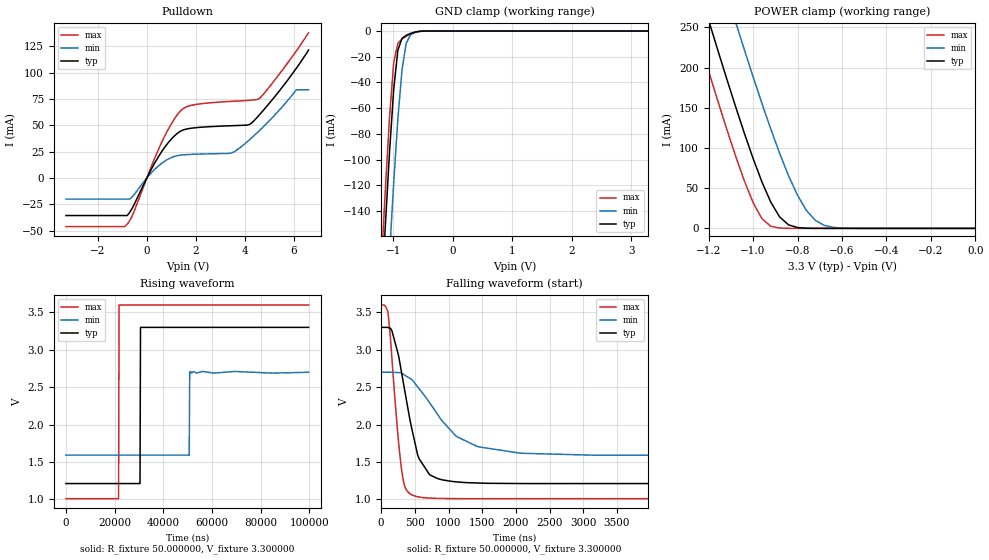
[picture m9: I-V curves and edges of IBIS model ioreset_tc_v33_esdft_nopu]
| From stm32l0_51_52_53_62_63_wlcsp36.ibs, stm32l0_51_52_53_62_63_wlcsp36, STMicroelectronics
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|   Model ioreset_tc_v33_esdft_nopu
[Model]  ioreset_tc_v33_esdft_nopu
Model_type I/O_open_drain
Polarity   Inverting
Enable   Active-High
Vinl =   0.990000V
Vinh =   2.310000V
Vmeas =  1.650000V
Cref =   1.0000000000000001E-7F
Rref =   1.000000k
Vref =   3.300000V
C_comp   1.946100pF   1.923200pF   1.977700pF
[Temperature Range]   25.000000   0.125000k   -40.000000
[Pullup Reference]   3.300000V   2.700000V   3.600000V
[Pulldown Reference]   0.0V   0.0V   0.0V
[POWER Clamp Reference]   3.300000V   2.700000V   3.600000V
[GND Clamp Reference]   0.0V   0.0V   0.0V
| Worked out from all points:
|   slope of the pulldown table from 0 to 0.495 V, typ, clamps not added: 23.6 ohm
|   GND clamp passes 1 mA (typ) near -0.65 V on its own axis
|   POWER clamp passes 1 mA (typ) near -0.80 V on its own axis
|   rising waveform, R_fixture 50.000000, V_fixture 3.300000: 20-80 % time 120ns typ, 119ns min, 120ns max; typ from 1.21 V to 3.3 V
|   falling waveform, R_fixture 50.000000, V_fixture 3.300000: 20-80 % time 267ns typ, 617ns min, 142ns max; typ from 3.3 V to 1.21 V
[Pulldown]
|Voltage   I(typ)   I(min)   I(max)
-3.3V     -35.57mA   -19.98mA   -46.06mA
-900mV    -35.57mA   -19.98mA   -46.06mA
-600mV    -28.81mA   -18.01mA   -36.04mA
600mV     24.81mA    13.84mA    33.52mA
1V        36.95mA    19.4mA     51.38mA
1.4V      44.71mA    21.77mA    64.22mA
1.9V      47.49mA    22.51mA    69.34mA
3.4V      49.55mA    23.44mA    72.65mA
4.2V      50.88mA    36.54mA    73.75mA
4.7V      62.76mA    47.3mA     77.96mA
6.1V      104.1mA    83.7mA     120.5mA
6.6V      121.4mA    83.7mA     137.7mA
[GND_clamp]
|Voltage   I(typ)   I(min)   I(max)
-3.3V     -2.25A     -2.322A    -2.233A
-1.2V     -211.8mA   -294.7mA   -184.2mA
-1.13V    -151mA     -233.2mA   -123.1mA
-1.06V    -94.15mA   -173.8mA   -67.07mA
-990mV    -45.49mA   -118mA     -24.73mA
-920mV    -14.87mA   -68.31mA   -9.524mA
-850mV    -5.685mA   -30.05mA   -6.27mA
-780mV    -3.335mA   -9.528mA   -4.082mA
-710mV    -1.932mA   -3.082mA   -2.278mA
-640mV    -914.4uA   -1.28mA    -971uA
-500mV    -57.12uA   -162.8uA   -33.58uA
3.28V     0A         0A         0A
[POWER_clamp]
|Voltage   I(typ)   I(min)   I(max)
-3.28V    2.284A     2.382A     2.228A
-1.28V    332.8mA    439.6mA    269.5mA
-1.24V    295.8mA    402.7mA    232.5mA
-1.2V     259.2mA    365.9mA    195.9mA
-1.16V    223.1mA    329.6mA    160mA
-1.08V    152.8mA    258mA      91.28mA
-960mV    57.8mA     155.4mA    12.02mA
-880mV    14.09mA    93.1mA     405uA
-800mV    1.048mA    41.21mA    11.87uA
-720mV    52.87uA    10.02mA    3.322uA
-600mV    2.856uA    415.9uA    1.64uA
0V        0A         0A         0A
[Ramp]
| variable   typ   min   max
dV/dt_r  1.25244/59.96266n   0.67104/61.04248n   1.55376/59.99537n
dV/dt_f  1.25244/0.29015u   0.66456/0.61907u   1.55376/0.15045u
R_load = 50.000000
[Rising Waveform]
R_fixture= 50.000000
V_fixture= 3.300000
V_fixture_min= 2.700000
V_fixture_max= 3.600000
|time   V(typ)   V(min)   V(max)
0s        1.213V     1.593V     1.01V
21.62us   1.213V     1.593V     1.01V
21.82us   1.213V     1.593V     3.6V
30.43us   1.211V     1.593V     3.6V
30.63us   3.3V       1.593V     3.6V
50.65us   3.3V       1.59V      3.6V
50.85us   3.3V       2.705V     3.6V
53.65us   3.3V       2.689V     3.6V
56.26us   3.3V       2.71V      3.6V
99.7us    3.3V       2.7V       3.6V
[Falling Waveform]
R_fixture= 50.000000
V_fixture= 3.300000
V_fixture_min= 2.700000
V_fixture_max= 3.600000
|time   V(typ)   V(min)   V(max)
0s        3.3V       2.7V       3.6V
100.1ns   3.299V     2.7V       3.509V
240.2ns   2.984V     2.697V     1.944V
320.3ns   2.607V     2.677V     1.292V
380.4ns   2.3V       2.644V     1.121V
520.5ns   1.68V      2.53V      1.041V
720.7ns   1.329V     2.291V     1.019V
1.121us   1.234V     1.84V      1.011V
2.062us   1.213V     1.619V     1.01V
9.97us    1.213V     1.593V     1.01V
